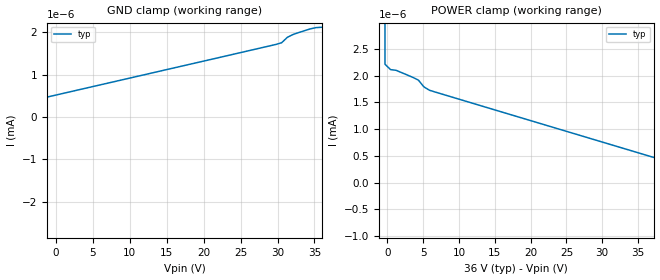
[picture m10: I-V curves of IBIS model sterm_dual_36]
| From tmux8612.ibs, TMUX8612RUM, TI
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| sterm_dual_36
[Model]   sterm_dual_36
Model_type   Terminator
|   typ   min   max
C_comp   6.362683e-12   NA   NA
[Voltage Range]   36   NA   NA
[Temperature Range]   27   NA   NA
[Power Clamp Reference]   36   NA   NA
[GND Clamp Reference]   0   NA   NA
[GND Clamp]
|   Voltage   I(typ)   I(min)   I(max)
-41V      -2.416A    NA         NA
-37.11V   -48.54mA   NA         NA
-36.33V   -2.01nA    NA         NA
-35.56V   -914.3pA   NA         NA
29.78V    1.715nA    NA         NA
30.56V    1.755nA    NA         NA
31.33V    1.884nA    NA         NA
32.11V    1.951nA    NA         NA
34.44V    2.083nA    NA         NA
36V       2.121nA    NA         NA
[POWER Clamp]
|   Voltage   I(typ)   I(min)   I(max)
-5V       1.055A     NA         NA
-1.111V   25.66mA    NA         NA
-333.3mV  2.217nA    NA         NA
444.4mV   2.116nA    NA         NA
1.222V    2.103nA    NA         NA
4.333V    1.919nA    NA         NA
5.111V    1.792nA    NA         NA
5.889V    1.729nA    NA         NA
72V       -932.4pA   NA         NA
